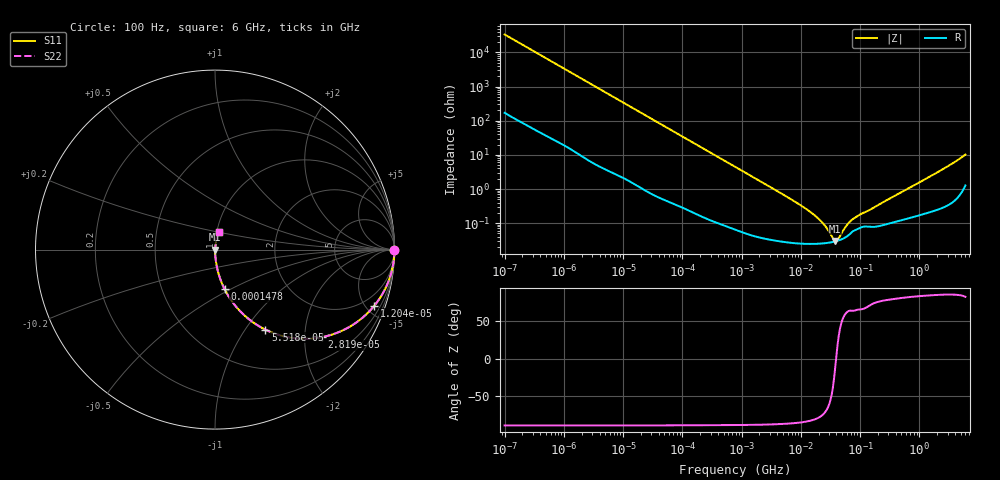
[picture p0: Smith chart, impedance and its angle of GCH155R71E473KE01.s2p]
!Murata Part Number: GCH155R71E473KE01
!These Parameters are Measured in Series Mode Connection
!Data Generated on Jun 19, 2026
!  o--ll--o
!Port1  Port2
!  o------o
!Operation Temp=25[degC], DC Bias Voltage=0[V]
!Freq. Start=100[Hz] Stop=6[GHz] 401[Steps]
# Hz S RI R 50
!Freq.(Hz) S11(Real) S11(Imag) S21(Real) S21(Imag) S12(Real) S12(Imag) S22(Real) S22(Imag)
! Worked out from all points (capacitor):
!   401 points, 100 Hz to 6 GHz, reference 50 ohm
!   read as one part in series: C = 47.3 nF near 109 Hz
!   lowest |Z| = 29.8 mohm at 38.09 MHz (marker M1)
!   series resonance near 39.44 MHz, so ESL is about 340 pH
!   S11 on the Smith chart (normalised r, x): 100 Hz: open; 12.04 kHz: 1.04, -5.67; 28.19 kHz: 1.02, -2.43; 55.18 kHz: 1.01, -1.24; 147.8 kHz: 1.00, -0.47; 6 GHz: 1.03, +0.20
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100  1 -0.00298  2.4e-05 0.00298  2.4e-05 0.00298  1 -0.00298
2008  0.9962 -0.0589  0.0038 0.0589  0.0038 0.0589  0.9962 -0.0589
5143  0.9769 -0.1475  0.0231 0.1475  0.0231 0.1475  0.9769 -0.1475
12041  0.8879 -0.3123  0.1121 0.3123  0.1121 0.3123  0.8879 -0.3123
18016  0.7815 -0.4101  0.2185 0.4101  0.2185 0.4101  0.7815 -0.4101
28191  0.5958 -0.4876  0.4042 0.4876  0.4042 0.4876  0.5958 -0.4876
40335  0.4203 -0.4903  0.5797 0.4903  0.5797 0.4903  0.4203 -0.4903
55182  0.2806 -0.4458  0.7194 0.4458  0.7194 0.4458  0.2806 -0.4458
86348  0.1391 -0.342  0.8609 0.342  0.8609 0.342  0.1391 -0.342
147774  0.0535 -0.2206  0.9465 0.2206  0.9465 0.2206  0.0535 -0.2206
316350  0.013 -0.108  0.987 0.108  0.987 0.108  0.013 -0.108
774597  0.00266 -0.0448  0.9973 0.0448  0.9973 0.0448  0.00266 -0.0448
6353432  0.000298 -0.00541  0.9997 0.00541  0.9997 0.00541  0.000298 -0.00541
1.555665e7  0.000251 -0.00192  0.9997 0.00192  0.9997 0.00192  0.000251 -0.00192
2.434276e7  0.000257 -0.000901  0.9997 0.000901  0.9997 0.000901  0.000257 -0.000901
3.80911e7  0.000292 -6.24e-05  0.9997 6.24e-05  0.9997 6.24e-05  0.000292 -6.24e-05
4.165952e7  0.000305 9.86e-05  0.9997 -9.86e-05  0.9997 -9.86e-05  0.000305 9.86e-05
5.960426e7  0.000406 0.000763  0.9996 -0.000763  0.9996 -0.000763  0.000406 0.000763
7.455971e7  0.000567 0.00117  0.9994 -0.00117  0.9994 -0.00117  0.000567 0.00117
3.124326e8  0.00101 0.00509  0.999 -0.00509  0.999 -0.00509  0.00101 0.00509
2.048624e9  0.00344 0.031  0.9966 -0.031  0.9966 -0.031  0.00344 0.031
6e9  0.0224 0.0983  0.9776 -0.0983  0.9776 -0.0983  0.0224 0.0983
